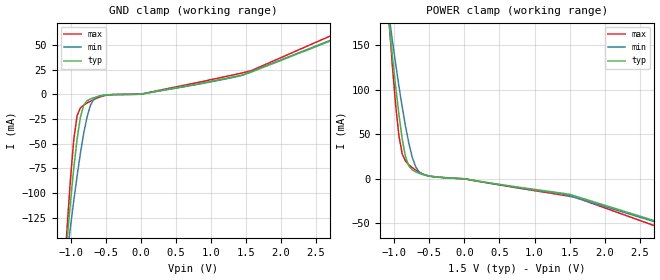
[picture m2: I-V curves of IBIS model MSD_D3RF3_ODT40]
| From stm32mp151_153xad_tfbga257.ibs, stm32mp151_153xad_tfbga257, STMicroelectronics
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[Model] MSD_D3RF3_ODT40
Model_type   Input
C_comp 2.139pF   2.100pF   2.210pF
Vinh = 925.000mV
Vinl = 575.000mV
[Temperature Range]   25.000   125.000   -40.000
[Voltage Range]   1.500V   1.425V   1.575V
[GND Clamp Reference]   0.00V   0.00V   0.00V
[POWER Clamp Reference]   1.500V   1.425V   1.575V
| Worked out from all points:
|   GND clamp passes 1 mA (typ) near -0.51 V on its own axis
|   POWER clamp passes 1 mA (typ) near -0.23 V on its own axis
[GND Clamp]
-1.48V    -548.9mA   -435.2mA   -711mA
-1.05V    -148.2mA   -163mA     -136mA
-1.002V   -110mA     -135mA     -86.63mA
-954.6mV  -75.25mA   -108.1mA   -46.26mA
-906.8mV  -45.42mA   -82.85mA   -21.84mA
-859.1mV  -23.04mA   -59.64mA   -13.72mA
-763.6mV  -6.52mA    -22.63mA   -8.912mA
-715.9mV  -4.74mA    -11.14mA   -7.07mA
-620.5mV  -2.6mA     -2.542mA   -3.866mA
900nV     12.29nA    11.63nA    13.94nA
1.575V    22.42mA    22.84mA    23.83mA
2.959V    61.05mA    61.81mA    66.98mA
[Power Clamp]
-1.459V   520.7mA    423.1mA    659.6mA
-1.077V   177.2mA    184.7mA    180.3mA
-1.03V    139.8mA    156.8mA    129.4mA
-981.8mV  104.6mA    129.9mA    83.68mA
-934.1mV  72.2mA     104.2mA    48.13mA
-886.4mV  44.32mA    80.23mA    27.77mA
-838.6mV  24.26mA    58.39mA    19.65mA
-743.2mV  10.06mA    23.98mA    12.6mA
-647.7mV  6.222mA    7.919mA    7.548mA
-552.3mV  3.866mA    4.048mA    4.125mA
1.548V    -18.62mA   -20.33mA   -20.29mA
2.98V     -53.72mA   -54.71mA   -60.33mA
